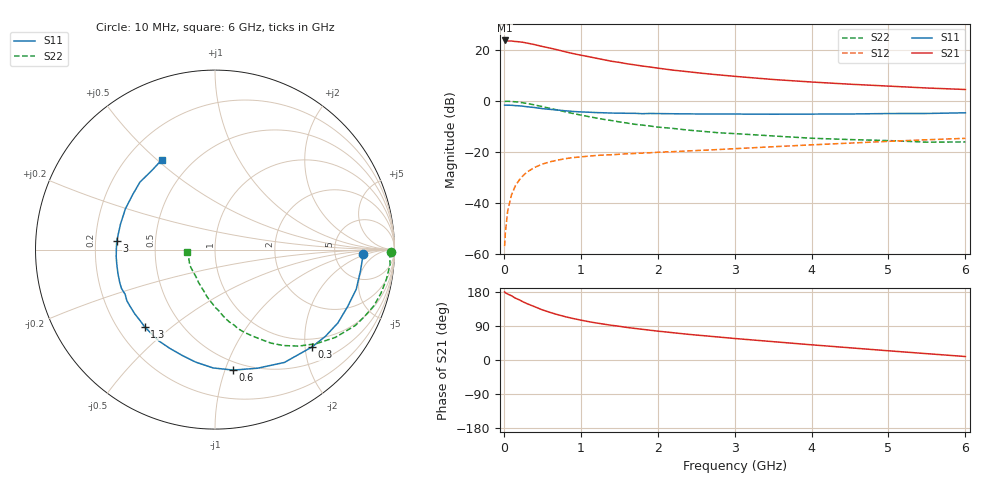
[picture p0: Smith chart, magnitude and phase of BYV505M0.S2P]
! SIEMENS Small Signal Semiconductors
! BFY420
! Si NPN RF SIEGET Grounded Emitter Transistor in MICRO-X
! VCE = 0.5 V  IC = 5 mA
! Common Emitter S-Parameters:  October  1996
# GHz  S  MA  R  50
!  f  S11  S21  S12  S22
! GHz  MAG  ANG  MAG  ANG  MAG  ANG  MAG  ANG
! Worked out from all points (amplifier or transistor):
!   36 points, 10 MHz to 6 GHz, reference 50 ohm
!   highest |S21| = 23.7 dB at 10 MHz (marker M1)
!   |S21| within 3 dB of that: start of sweep to 600.3 MHz
!   unconditionally stable (mu >= 1): 2.95 GHz to end of sweep
!   at 250 MHz: K = 0.12, MSG = 26.2 dB, |S12| = -29.4 dB
!   at 1.4 GHz: K = 0.57, MSG = 18.4 dB, |S12| = -21.2 dB
!   at 6 GHz: K = 1.18, MAG = 7.0 dB, |S12| = -14.7 dB
!   S11 on the Smith chart (normalised r, x): 10 MHz: 10, -1; 300 MHz: 0.82, -2.14; 600 MHz: 0.43, -1.07; 1.3 GHz: 0.31, -0.41; 3 GHz: 0.29, +0.04; 6 GHz: 0.34, +0.52
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0.01  0.8225 -1.6  15.3 179.8  0.0014 100.0  0.9821 -0.9
0.02  0.8231 -3.6  15.3 177.4  0.0026 92.1  0.9747 -1.9
0.05  0.8195 -8.0  14.92 174.1  0.0069 88.1  0.9787 -4.9
0.1  0.8174 -15.7  14.93 169.5  0.0143 83.2  0.969 -9.9
0.15  0.8043 -23.2  14.59 163.2  0.0215 76.5  0.956 -14.8
0.2  0.7974 -30.8  14.4 158.9  0.0278 73.9  0.9394 -19.4
0.25  0.7823 -38.2  14.07 153.5  0.034 69.3  0.9132 -24.0
0.3  0.7654 -45.2  13.61 148.8  0.0398 66.8  0.8897 -28.3
0.4  0.7381 -58.4  12.69 140.7  0.0492 59.9  0.8302 -36.1
0.5  0.702 -70.3  11.66 132.3  0.0572 53.9  0.7693 -43.0
0.6  0.679 -81.4  10.84 125.7  0.0635 50.0  0.7113 -49.1
0.8  0.6364 -99.6  9.165 114.2  0.0732 42.5  0.6071 -59.1
0.9  0.6179 -107.0  8.457 109.5  0.0767 40.1  0.563 -62.8
1.1  0.5976 -121.5  7.369 101.3  0.0819 36.3  0.4908 -70.3
1.3  0.5819 -132.3  6.407 94.6  0.0862 33.2  0.4317 -76.0
1.7  0.5676 -149.9  5.079 83.4  0.0925 30.2  0.3465 -85.8
2.2  0.5571 -166.1  3.998 72.0  0.1005 27.9  0.287 -95.5
3  0.5495 175.0  3.024 56.8  0.1148 25.9  0.2271 -108.7
3.5  0.5454 164.9  2.621 48.4  0.1254 24.5  0.2041 -116.8
4.5  0.5512 146.6  2.118 32.2  0.1479 19.6  0.1734 -134.4
5.5  0.5639 128.7  1.784 16.7  0.1718 13.1  0.1541 -161.1
6  0.5817 120.6  1.668 9.2  0.1834 9.6  0.1558 -175.9
